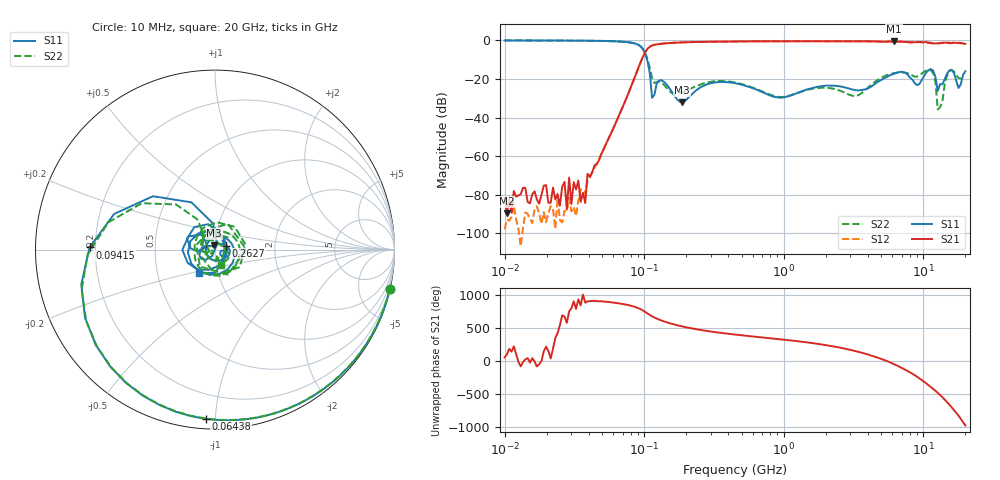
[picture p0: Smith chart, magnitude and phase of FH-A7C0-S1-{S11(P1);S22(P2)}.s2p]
!Agilent Technologies,N5230A,MY45001737,A.07.50.48
!Agilent N5230A: A.07.50.48
!Date: Friday, August 09, 2024 17:49:14
!Correction: S22(Full 2 Port(2,4))
!S42(Full 2 Port(2,4))
!S24(Full 2 Port(2,4))
!S44(Full 2 Port(2,4))
!S2P File: Measurements: S22, S42, S24, S44:Log Frequency Sweep
# Hz S  MA  R 50
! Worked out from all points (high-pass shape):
!   201 points, 10 MHz to 20 GHz, reference 50 ohm
!   highest |S21| = -0.41 dB at 6.157 GHz (marker M1); lowest = -89.6 dB at 10.39 MHz (marker M2)
!   |S21| within 3 dB of the highest: 109.1 MHz to end of sweep
!   lowest |S11| = -32.1 dB at 186.6 MHz (marker M3), VSWR 1.05, Z = 49.4 + j2.41 ohm
!   |S11| at or under -10 dB: 104.9 MHz to end of sweep
!   |S22| runs from -35.8 to 0.0 dB; largest |S21 - S12| = 0.043
!   S11 on the Smith chart (normalised r, x): 10 MHz: 0.05, -9.10; 64.38 MHz: 0.05, -0.94; 94.15 MHz: 0.18, +0.01; 262.7 MHz: 1.13, +0.05; 20 GHz: 0.81, -0.22
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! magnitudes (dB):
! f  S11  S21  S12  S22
! 10 MHz  0.0  -81.6  -97.8  0.0
! 10.39 MHz  0.0  -89.6  -92.7  0.0
! 27.9 MHz  -0.1  -87.6  -88.6  -0.1
! 28.98 MHz  -0.1  -71.0  -81.5  -0.1
! 36.41 MHz  -0.1  -79.0  -80.3  -0.1
! 64.38 MHz  -0.5  -40.8  -40.7  -0.5
! 94.15 MHz  -3.1  -11.3  -11.3  -3.0
! 105.5 MHz  -10.6  -4.4  -4.4  -9.6
! 113.8 MHz  -29.7  -2.6  -2.6  -19.4
! 127.6 MHz  -20.7  -1.9  -1.9  -21.4
! 186.6 MHz  -32.1  -1.0  -1.0  -26.8
! 262.7 MHz  -23.7  -0.7  -0.7  -22.4
! 447.2 MHz  -22.1  -0.5  -0.5  -21.8
! 1.628 GHz  -24.5  -0.4  -0.4  -24.9
! 3.352 GHz  -25.8  -0.5  -0.4  -28.6
! 5.706 GHz  -18.2  -0.5  -0.5  -17.5
! 6.157 GHz  -17.2  -0.4  -0.6  -17.0
! 11.31 GHz  -14.8  -1.4  -1.2  -15.4
! 12.68 GHz  -26.2  -1.5  -1.5  -35.8
! 15.33 GHz  -15.5  -1.4  -1.2  -15.9
! 17.84 GHz  -24.7  -1.2  -1.4  -19.4
! 20 GHz  -16.0  -1.7  -1.9  -20.5
